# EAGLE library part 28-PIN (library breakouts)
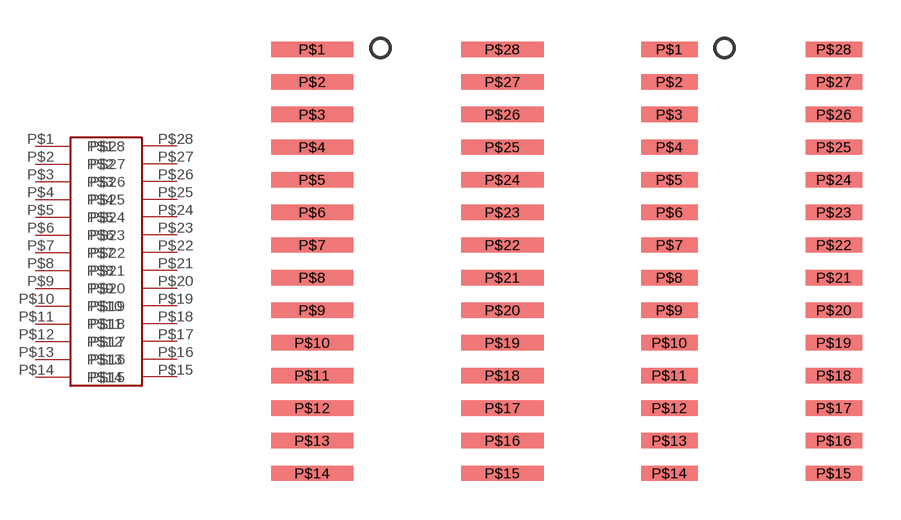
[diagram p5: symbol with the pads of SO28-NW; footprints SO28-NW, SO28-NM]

Designator prefix -

## 28-PINSOIC-NW  [SO28-NW]
P$1  P$1
P$2  P$2
P$3  P$3
P$4  P$4
P$5  P$5
P$6  P$6
P$7  P$7
P$8  P$8
P$9  P$9
P$10  P$10
P$11  P$11
P$12  P$12
P$13  P$13
P$14  P$14
P$15  P$15
P$16  P$16
P$17  P$17
P$18  P$18
P$19  P$19
P$20  P$20
P$21  P$21
P$22  P$22
P$23  P$23
P$24  P$24
P$25  P$25
P$26  P$26
P$27  P$27
P$28  P$28

## 28-PINSOIC-NM  [SO28-NM]
Pads as for SO28-NW

## 28-PINSOIC-M  [SO28-M]
Pads as for SO28-NW

## 28-PINTSSOP-N  [TSSOP28-3.9]
Pads as for SO28-NW

## 28-PINSOIC-N  [SO28-N]
Pads as for SO28-NW

## 28-PINSOIC-MW  [SO28-MW]
Pads as for SO28-NW

## 28-PINSOIC-W  [SO28-W]
Pads as for SO28-NW

## 28-PINTSSOP-W  [TSSOP28-5.3]
Pads as for SO28-NW

## 28-PINTSSOP-NW  [TSSOP28-NW]
Pads as for SO28-NW

## Footprint SO28-NW (pad centres in mm)
smd 3.2 x 0.6: P$1 -3.7,8.255; P$2 -3.7,6.985; P$3 -3.7,5.715; P$4 -3.7,4.445; P$5 -3.7,3.175; P$6 -3.7,1.905; P$7 -3.7,0.635; P$8 -3.7,-0.635; P$9 -3.7,-1.905; P$10 -3.7,-3.175; P$11 -3.7,-4.445; P$12 -3.7,-5.715; P$13 -3.7,-6.985; P$14 -3.7,-8.255; P$15 3.7,-8.255; P$16 3.7,-6.985; P$17 3.7,-5.715; P$18 3.7,-4.445; P$19 3.7,-3.175; P$20 3.7,-1.905; P$21 3.7,-0.635; P$22 3.7,0.635; P$23 3.7,1.905; P$24 3.7,3.175; P$25 3.7,4.445; P$26 3.7,5.715; P$27 3.7,6.985; P$28 3.7,8.255

## Footprint SO28-NM (pad centres in mm)
smd 2.2 x 0.6: P$1 -3.2,8.255; P$2 -3.2,6.985; P$3 -3.2,5.715; P$4 -3.2,4.445; P$5 -3.2,3.175; P$6 -3.2,1.905; P$7 -3.2,0.635; P$8 -3.2,-0.635; P$9 -3.2,-1.905; P$10 -3.2,-3.175; P$11 -3.2,-4.445; P$12 -3.2,-5.715; P$13 -3.2,-6.985; P$14 -3.2,-8.255; P$15 3.2,-8.255; P$16 3.2,-6.985; P$17 3.2,-5.715; P$18 3.2,-4.445; P$19 3.2,-3.175; P$20 3.2,-1.905; P$21 3.2,-0.635; P$22 3.2,0.635; P$23 3.2,1.905; P$24 3.2,3.175; P$25 3.2,4.445; P$26 3.2,5.715; P$27 3.2,6.985; P$28 3.2,8.255

## Footprint SO28-M (pad centres in mm)
smd 1.2 x 0.6: P$1 -3.7,8.255; P$2 -3.7,6.985; P$3 -3.7,5.715; P$4 -3.7,4.445; P$5 -3.7,3.175; P$6 -3.7,1.905; P$7 -3.7,0.635; P$8 -3.7,-0.635; P$9 -3.7,-1.905; P$10 -3.7,-3.175; P$11 -3.7,-4.445; P$12 -3.7,-5.715; P$13 -3.7,-6.985; P$14 -3.7,-8.255; P$15 3.7,-8.255; P$16 3.7,-6.985; P$17 3.7,-5.715; P$18 3.7,-4.445; P$19 3.7,-3.175; P$20 3.7,-1.905; P$21 3.7,-0.635; P$22 3.7,0.635; P$23 3.7,1.905; P$24 3.7,3.175; P$25 3.7,4.445; P$26 3.7,5.715; P$27 3.7,6.985; P$28 3.7,8.255

## Footprint TSSOP28-3.9 (pad centres in mm)
smd 1.4 x 0.35: P$1 -2.65,4.225; P$2 -2.65,3.575; P$3 -2.65,2.925; P$4 -2.65,2.275; P$5 -2.65,1.625; P$6 -2.65,0.975; P$7 -2.65,0.325; P$8 -2.65,-0.325; P$9 -2.65,-0.975; P$10 -2.65,-1.625; P$11 -2.65,-2.275; P$12 -2.65,-2.925; P$13 -2.65,-3.575; P$14 -2.65,-4.225; P$15 2.65,-4.225; P$16 2.65,-3.575; P$17 2.65,-2.925; P$18 2.65,-2.275; P$19 2.65,-1.625; P$20 2.65,-0.975; P$21 2.65,-0.325; P$22 2.65,0.325; P$23 2.65,0.975; P$24 2.65,1.625; P$25 2.65,2.275; P$26 2.65,2.925; P$27 2.65,3.575; P$28 2.65,4.225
